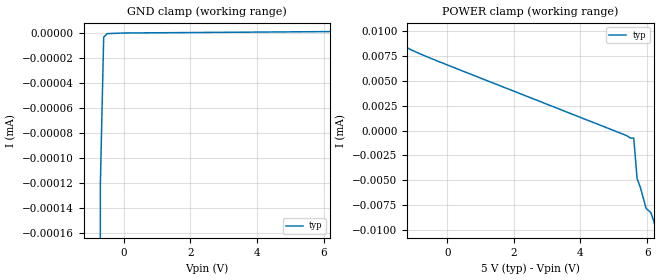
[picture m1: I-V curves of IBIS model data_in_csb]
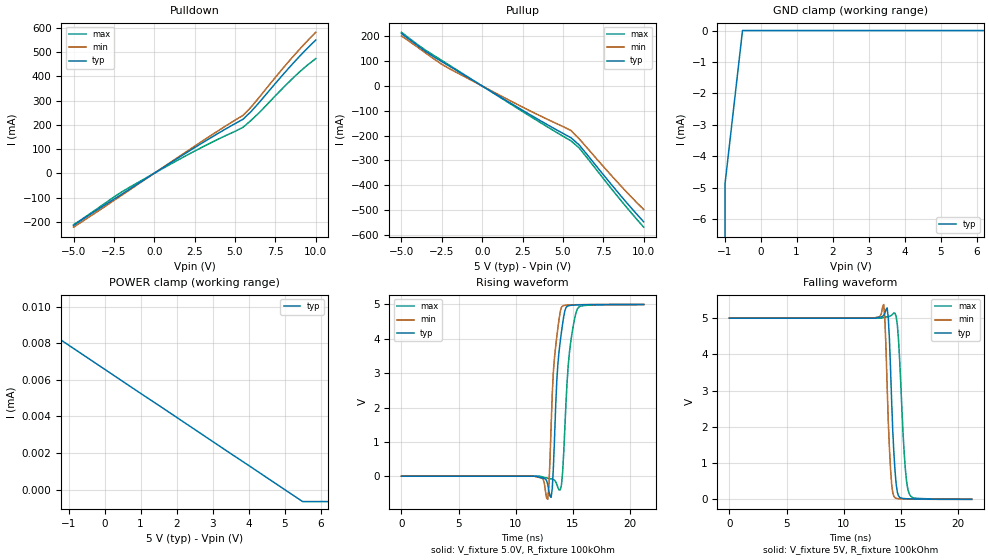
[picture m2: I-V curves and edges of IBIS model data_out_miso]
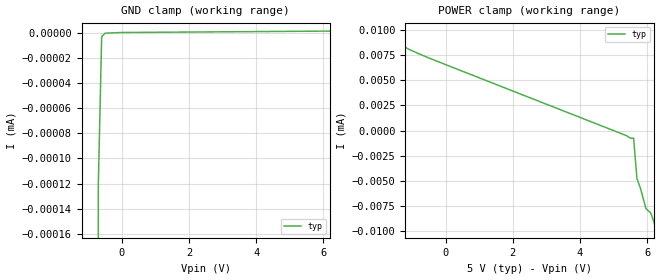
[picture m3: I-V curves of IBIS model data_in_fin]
[IBIS Ver]   4.0
[File name]   fs8500.ibs
[File Rev]   1.0
[Date]   June 2019
[Source]   NXP semiconductors
[Notes]   IBIS model for the FS8500 includes the model of SPI pins
|   (SCLK. CSB. MOSI and MISO).
|   I2C pins SCL and SDA) and FIN.FOUT at 5.0V
[Disclaimer]   This information is for modeling purposes only
|   and is not guaranteed.The simulation model is not able to
|   reproduce identically the quality structure
|   and behavior of the final product.
[Copyright]   Copyright 2019 NXP Semiconductors: All Rights Reserved. This
|   simulation model or derivative thereof is the proprietary
|   information of NXP Semiconductors. is confidential in nature
|   and may not be reproduced in any way
|   (physically or electronically)
|   without the express permission from NXP Semiconductors.
[Component]   fs8500
[Manufacturer]   NXP semiconductors
[Package]
|   typ   min   max
R_pkg   0.098245   0.052042   0.124
L_pkg   2.342e-9   1.324e-9   2.878e-9
C_pkg   4.62e-13   3.4e-13   8.59e-13
[Pin]   Signal_name   model_name   R_pin   L_pin   C_pin
4   VDDI2C   POWER
23   VDDIO   POWER
29   AMUX   NC   0.1134   2.75e-9   4.516e-13
5   BOOST_LS   NC   0.052042   1.324e-9   6.306e-13
39   BUCK1_FB   NC   0.10342   2.436e-9   3.779e-13
36   BUCK1_IN   NC   0.053399   1.436e-9   8.465e-13
37   BUCK1_SW   NC   0.054528   1.462e-9   8.037e-13
32   BUCK2_FB   NC   0.10292   2.413e-9   3.775e-13
35   BUCK2_IN   NC   0.053731   1.431e-9   8.59e-13
34   BUCK2_SW   NC   0.055152   1.442e-9   8.438e-13
9   BUCK3_FB   NC   0.10164   2.274e-9   3.452e-13
6   BUCK3_IN   NC   0.052811   1.38e-9   7.746e-13
3   BUCK3_INQ   NC   0.10905   2.09e-9   3.719e-13
7   BUCK3_SW   NC   0.052819   1.374e-9   7.814e-13
28   CSB   data_in_csb   0.11755   2.815e-9   4.599e-13
8   DBG   NC   0.1024   2.286e-9   3.421e-13
40   ERRMON   NC   0.10613   2.518e-9   4.14e-13
31   FCCU1   NC   0.10522   2.517e-9   4.116e-13
30   FCCU2   NC   0.10909   2.635e-9   4.281e-13
20   FIN   data_in_fin   0.10609   2.451e-9   3.713e-13
24   FOUT   data_out_fout   0.10662   2.265e-9   3.668e-13
14   FS0B   NC   0.11495   2.78e-9   4.562e-13
22   GND   NC   0.069511   1.692e-9   4.64e-13
21   GNDFS   NC   0.068844   1.855e-9   4.551e-13
33   INTB   NC   0.10157   2.282e-9   3.647e-13
55   LDO1   NC   0.075736   2.24e-9   5.233e-13
56   LDO1_IN   NC   0.12263   2.875e-9   4.573e-13
54   LDO2   NC   0.075013   2.208e-9   5.166e-13
25   MISO   data_out_miso   0.10712   2.442e-9   3.922e-13
26   MOSI   data_in_mosi   0.11011   2.589e-9   4.246e-13
18   PGOOD   NC   0.10956   2.624e-9   3.883e-13
46   PRE_BOOT   NC   0.10905   2.575e-9   3.928e-13
41   PRE_COMP   NC   0.11161   2.64e-9   4.271e-13
42   PRE_CSP   NC   0.12009   2.722e-9   4.637e-13
48   PRE_FB   NC   0.1092   2.427e-9   3.737e-13
45   PRE_GHS   NC   0.11167   2.668e-9   4.246e-13
43   PRE_GLS   NC   0.124   2.77e-9   4.723e-13
44   PRE_SW   NC   0.11475   2.709e-9   4.347e-13
38   PSYNC   NC   0.10106   2.385e-9   3.473e-13
19   RSTB   NC   0.10602   2.512e-9   3.751e-13
10   SCL   data_in_scl   0.10255   2.333e-9   3.612e-13
27   SCLK   data_in_sclk   0.11237   2.691e-9   4.328e-13
11   SDA   data_in_out_sda  0.10245   2.418e-9   3.805e-13
53   VBOOST   NC   0.11134   2.667e-9   3.691e-13
47   VBOS   NC   0.070983   1.972e-9   4.536e-13
17   VCOREMON   NC   0.11098   2.683e-9   4.12e-13
16   VMON1   NC   0.11374   2.766e-9   4.209e-13
15   VMON2   NC   0.11882   2.878e-9   4.45e-13
13   VMON3   NC   0.10717   2.601e-9   4.195e-13
12   VMON4   NC   0.1042   2.489e-9   4.064e-13
50   VSUP1   NC   0.10369   2.455e-9   3.727e-13
51   VSUP2   NC   0.10511   2.516e-9   3.4e-13
49   WAKE1   NC   0.10447   2.442e-9   3.702e-13
1   WAKE2   NC   0.12036   2.577e-9   4.265e-13
2   EP   GND
| end pin list
| Models and submodels in the file (8): data_in_csb (Input), data_in_sclk (Input), data_in_mosi (Input), data_out_miso (Output), data_in_fin (Input), data_out_fout (Output), data_in_scl (Input), data_in_out_sda (I/O_open_drain)
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|   Model data_in_csb
[Model]   data_in_csb
Model_type   Input
Polarity   Non-Inverting
|   typ   min   max
C_comp   79.83f   69.66f   104.6f
| Where typ is typical value of c_comp (no PVT)
|   min is the minimum value of c_comp under PVT
|   max is the maximum value of c_comp under PVT
Vinh  =   3.053
Vinl  =   1.87
| Hysteresis
|   |   Rising Edge   Falling Edge
|   |   Switching Region   oo   o   Switching Region
|   |   |  o   oo  ooooooooo   |
|   |   V o   o   |
| Vinh  - - - - - - - - - - x   o   |
|   |   o   o  |
|   |   o   o |
|   |   o   oV
| Vinl  - - - - - - -  o - - - - - - - - - - - - - - - - - x
|   |   o   o
|   |   o   o
|   |oooooo-----------------------------------------------------oooooooo
|   typ min max
[Power Clamp Reference]  5.0 NA NA
[GND Clamp Reference]   0   NA NA
[pullup reference]   5.0 NA NA
[pulldown reference]   0   NA NA
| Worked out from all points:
|   POWER clamp passes 1 mA (typ) near -2.32 V on its own axis
[GND Clamp]
|Voltage   I(typ)   I(min)   I(max)
-5V       -4A        NA         NA
-1.006V   -9.4mA     NA         NA
-700mV    -121nA     NA         NA
-600mV    -3.33nA    NA         NA
-500mV    -562pA     NA         NA
10V       1.59nA     NA         NA
[POWER Clamp]
|Voltage   I(typ)   I(min)   I(max)
-5V       2A         NA         NA
-1.5V     12.6uA     NA         NA
-1.3V     8.66uA     NA         NA
-1.1V     8.12uA     NA         NA
5.6V      -761nA     NA         NA
5.7V      -4.82uA    NA         NA
5.8V      -5.72uA    NA         NA
5.97V     -7.81uA    NA         NA
6.111V    -8.23uA    NA         NA
6.204V    -9.11uA    NA         NA
6.307V    -10.5uA    NA         NA
10V       -15uA      NA         NA
|   Model data_out_miso
[Model]   data_out_miso
Model_type   Output
Polarity   Non-Inverting
Vmeas = 2.5
Cref = 0pF
Rref = 50
|   typ   min   max
C_comp   2.949p  2.447p  4.788p
|   typ min max
[Power Clamp Reference]  5.0 NA NA
[GND Clamp Reference]   0   NA NA
[pullup reference]   5.0 NA NA
[pulldown reference]   0   NA NA
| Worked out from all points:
|   slope of the pulldown table from 0 to 0.75 V, typ, clamps not added: 23.4 ohm
|   slope of the pullup table from 0 to 0.75 V, typ, clamps not added: 25.4 ohm
|   rising waveform, V_fixture 5.0V, R_fixture 100kOhm: 20-80 % time 541ps typ, 522ps min, 611ps max; typ from 0.001 V to 5 V
|   falling waveform, V_fixture 5V, R_fixture 100kOhm: 20-80 % time 396ps typ, 356ps min, 488ps max; typ from 5 V to 0.001 V
[GND Clamp]
|Voltage   I(typ)   I(min)   I(max)
-5V       -4.5A      NA         NA
-1.267V   -210mA     NA         NA
-984mV    -4.86mA    NA         NA
-500mV    -562pA     NA         NA
10V       909pA      NA         NA
[POWER Clamp]
|Voltage   I(typ)   I(min)   I(max)
-5V       3A         NA         NA
-2.42V    505uA      NA         NA
-1.944V   9.14uA     NA         NA
5.5V      -658nA     NA         NA
10V       -658nA     NA         NA
|   typ   min   max
[Temperature Range]   27   -40   175
[Pulldown]
|Voltage   I(typ)   I(min)   I(max)
-5V       -215.6mA   -222.2mA   -212.3mA
-2.5V     -107mA     -112.4mA   -98.17mA
-1.5V     -64.38mA   -67.47mA   -56.74mA
2.5V      105.7mA    111.6mA    91.32mA
5.5V      222.8mA    238.8mA    189.5mA
6V        254.8mA    273.1mA    218.4mA
6.5V      291.9mA    313.1mA    249.8mA
8.5V      446.2mA    474mA      386.7mA
9.5V      516.7mA    547.1mA    446.9mA
10V       549.2mA    581.1mA    472.6mA
[Pullup]
|Voltage   I(typ)   I(min)   (max)
-5V       211.3mA    201.9mA    216.4mA
-3.5V     138.9mA    132.9mA    144mA
-2.5V     98.27mA    87.25mA    103mA
-2V       78.76mA    68.74mA    82.5mA
2.5V      -97.85mA   -84.92mA   -102.8mA
5.5V      -208.5mA   -179.5mA   -221.1mA
6V        -237.1mA   -212.5mA   -249.3mA
8.5V      -436mA     -396.4mA   -454mA
10V       -547.1mA   -497.5mA   -568.8mA
[Ramp]
R_load = 100kohm
|   typ   min   max
dV/dt_r   4.955/1e-9   4.277/1e-9   5.236/1e-9
dV/dt_f   6.882/1e-9   5.485/1e-9   7.724/1e-9
[Rising Waveform]
V_fixture = 5.0V
R_fixture = 100kOhm
|Time   V(typ)   V(min)   V(max)
0s        1.16mV     1.11mV     1.32mV
12.8ns    -237mV     -672mV     -56.9mV
13.1ns    -614mV     1.47V      -76.8mV
13.4ns    1.14V      3.473V     -116mV
13.6ns    2.814V     4.072V     -237mV
14ns      4.192V     4.915V     -259mV
14.4ns    4.911V     4.979V     2.14V
14.8ns    4.975V     4.989V     3.873V
15.5ns    4.989V     4.994V     4.917V
21.2ns    5V         5V         4.999V
[falling Waveform]
V_fixture = 5V
R_fixture = 100kOhm
|Time   V(typ)   V(min)   V(max)
0s        5V         5V         5V
13.5ns    5.08V      5.379V     5.02V
13.6ns    5.133V     5.013V     5.028V
13.9ns    5.033V     2.18V      5.042V
14.2ns    2.692V     418mV      5.087V
14.4ns    1.25V      80.5mV     5.147V
14.7ns    196mV      22.2mV     4.804V
15.3ns    22mV       11.2mV     1.264V
15.7ns    15.4mV     8.15mV     187mV
21.2ns    1.23mV     1.13mV     2.53mV
|   Model data_in_fin
[Model]   data_in_fin
Model_type   Input
Polarity   Non-Inverting
|   typ   min   max
C_comp   82.93f   66.37f   93.58f
| Where typ is typical value of c_comp (no PVT)
|   min is the minimum value of c_comp under PVT
|   max is the maximum value of c_comp under PVT
Vinh  =   2.327
Vinl  =   2.132
| Hysteresis
|   |   Rising Edge   Falling Edge
|   |   Switching Region   oo   o   Switching Region
|   |   |  o   oo  ooooooooo   |
|   |   V o   o   |
| Vinh  - - - - - - - - - - x   o   |
|   |   o   o  |
|   |   o   o |
|   |   o   oV
| Vinl  - - - - - - -  o - - - - - - - - - - - - - - - - - x
|   |   o   o
|   |   o   o
|   |oooooo-----------------------------------------------------oooooooo
|   typ min max
[Power Clamp Reference]  5.0 NA NA
[GND Clamp Reference]   0   NA NA
[pullup reference]   5.0 NA NA
[pulldown reference]   0   NA NA
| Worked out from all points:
|   POWER clamp passes 1 mA (typ) near -2.32 V on its own axis
[GND Clamp]
|Voltage   I(typ)   I(min)   I(max)
-5V       -4A        NA         NA
-1.006V   -9.4mA     NA         NA
-700mV    -121nA     NA         NA
-600mV    -3.33nA    NA         NA
-500mV    -562pA     NA         NA
10V       1.59nA     NA         NA
[POWER Clamp]
|Voltage   I(typ)   I(min)   I(max)
-5V       2A         NA         NA
-1.5V     12.6uA     NA         NA
-1.3V     8.66uA     NA         NA
-1.1V     8.12uA     NA         NA
5.6V      -761nA     NA         NA
5.7V      -4.82uA    NA         NA
5.8V      -5.72uA    NA         NA
5.97V     -7.81uA    NA         NA
6.111V    -8.23uA    NA         NA
6.204V    -9.11uA    NA         NA
6.307V    -10.5uA    NA         NA
10V       -15uA      NA         NA
